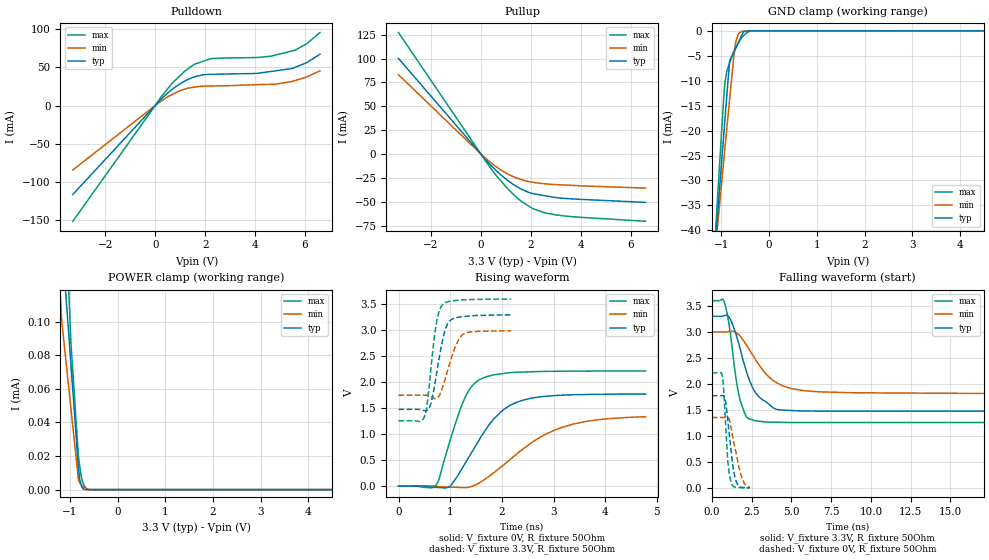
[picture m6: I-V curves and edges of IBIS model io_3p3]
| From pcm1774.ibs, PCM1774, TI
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|   io_3p3 Model
[Model]   io_3p3
Model_type   I/O
Polarity   Non-Inverting
Enable   Active-Low
Vinl = 0.99
Vinh = 2.31
Vmeas = 1.65
Vref = 1.65
Cref = 10pF
Rref = 50
|   typ   min   max
|   (nom PVT)   (fast PVT)   (slow PVT)
C_comp   8.631e-13   8.443e-13   8.826e-13
|ON state : BUFFER OUTPUT TURNED HIGH
|C_comp   8.631e-13   8.443e-13   8.826e-13
|OFF state: BUFFER IN HIGH IMPEDANCE
|C_comp   8.663e-13   8.474e-13   8.760e-13
| Where nom  PVT is Nominal Process, 3.3V, 26C
|   Fast PVT is Strong Process,  3.6V, -40C
|   Slow PVT is Weak Process,   3V, 86C
[Model Spec]
|Subparameter   typ   min   max
Vinh   2.31   2.1   2.52
Vinl   0.99   0.9   1.08
[Voltage Range]   3.3   3   3.6
|Ambient Temperature   25   85   -40
|Junction Temperature
[Temperature Range]   26   86   -40
[Pullup Reference]   3.3   3   3.6
[Pulldown Reference]   0   0   0
[Power Clamp Reference]   3.3   3   3.6
[GND Clamp Reference]   0   0   0
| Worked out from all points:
|   slope of the pulldown table from 0 to 0.495 V, typ, clamps not added: 30.8 ohm
|   slope of the pullup table from 0 to 0.495 V, typ, clamps not added: 34.8 ohm
|   GND clamp passes 1 mA (typ) near -0.58 V on its own axis
|   POWER clamp passes 1 mA (typ) near -2.56 V on its own axis
|   falling waveform, V_fixture 3.3V, R_fixture 50Ohm: 20-80 % time 1.19ns typ, 2.04ns min, 657ps max; typ from 3.3 V to 1.48 V
|   rising waveform, V_fixture 0V, R_fixture 50Ohm: 20-80 % time 730ps typ, 1.15ns min, 453ps max; typ from 0 V to 1.77 V
|   rising waveform, V_fixture 3.3V, R_fixture 50Ohm: 20-80 % time 201ps typ, 244ps min, 160ps max; typ from 1.48 V to 3.29 V
|   falling waveform, V_fixture 0V, R_fixture 50Ohm: 20-80 % time 394ps typ, 553ps min, 260ps max; typ from 1.77 V to 0.003 V
[Pulldown]
|   Voltage   I(typ)   I(min)   I(max)
-3.3V     -116.5mA   -84.42mA   -151.6mA
271.2mV   9.421mA    6.375mA    12.76mA
714mV     22.1mA     15.03mA    30.35mA
1.355V    34.85mA    23mA       49.31mA
1.589V    37.79mA    24.19mA    54.3mA
1.917V    40.27mA    25.38mA    57.97mA
2.222V    40.84mA    25.66mA    61.38mA
4.138V    42.37mA    27.45mA    62.98mA
4.8V      45.41mA    28mA       66.04mA
5.606V    50.05mA    32.82mA    72.53mA
6.082V    56.53mA    37.71mA    81.29mA
6.6V      67.25mA    45.42mA    95.62mA
[GND Clamp]
|   Voltage   I(typ)   I(min)   I(max)
-3.3V     -316.9mA   -268mA     -391.9mA
-1.111V   -40.79mA   -42.24mA   -38.36mA
-1.018V   -29.09mA   -32.77mA   -23.56mA
-949.2mV  -20.65mA   -25.85mA   -13.18mA
-920.4mV  -17.15mA   -22.94mA   -10.06mA
-825mV    -5.93mA    -13.45mA   -6.269mA
-738mV    -4.2mA     -5.003mA   -4.306mA
-702mV    -3.484mA   -2.489mA   -3.5mA
-648mV    -2.41mA    -754uA     -2.54mA
-567mV    -798.9uA   -93.27uA   -1.299mA
-243.6mV  -1.294uA   -116.1nA   -293.8nA
6.6V      0A         0A         0A
[Pullup]
|   Voltage   I(typ)   I(min)   I(max)
-3.3V     100.1mA    83.05mA    127.2mA
3mV       -185.6uA   -161.8uA   -246.1uA
363mV     -10.77mA   -8.423mA   -13.7mA
638.4mV   -18mA      -13.71mA   -23.32mA
1.103V    -28.28mA   -21.31mA   -37.21mA
1.643V    -37.09mA   -26.87mA   -49.95mA
2.064V    -41.39mA   -29.49mA   -56.97mA
2.525V    -43.47mA   -31.08mA   -61.32mA
3.018V    -45.7mA    -32.05mA   -63.8mA
3.983V    -47.45mA   -33.25mA   -66.26mA
6.6V      -50.64mA   -35.68mA   -70.46mA
[POWER Clamp]
|   Voltage   I(typ)   I(min)   I(max)
-3.3V     2.453mA    1.841mA    2.082mA
-1.947V   666.7uA    483.9uA    905uA
-1.178V   152uA      103.5uA    226.7uA
-1.165V   147uA      98.22uA    216.4uA
-981.6mV  75.07uA    48.64uA    88.02uA
-822mV    12.95uA    5.545uA    19.56uA
-788.7mV  5.054uA    3.952uA    12.72uA
-765.6mV  2.875uA    2.846uA    7.967uA
-736.8mV  979nA      2.084uA    4.528uA
-706.2mV  0A         1.47uA     2.727uA
-614.4mV  0A         0A         31.31nA
6.6V      0A         0A         0A
[Ramp]
R_load = 50
|   typ   min   max
dV/dt_r   1.06378/7.29577e-10   0.812608/1.17719e-09   1.32828/4.52863e-10
dV/dt_f   1.09414/1.19156e-09   0.751811/2.05432e-09   1.40532/6.56827e-10
[Falling Waveform]
V_fixture = 3.3V
V_fixture_min = 3V
V_fixture_max = 3.6V
R_fixture = 50Ohm
|   Time   V(typ)   V(min)   V(max)
0s        3.3V       3V         3.6V
770.7ps   3.31V      3V         3.581V
1.174ns   3.234V     3.015V     2.947V
1.504ns   2.966V     2.996V     2.133V
1.763ns   2.69V      2.921V     1.703V
2.146ns   2.264V     2.76V      1.384V
2.666ns   1.872V     2.508V     1.296V
4.032ns   1.515V     2.03V      1.263V
6.027ns   1.48V      1.864V     1.258V
27.16ns   1.477V     1.751V     1.258V
[Rising Waveform]
V_fixture = 0V
V_fixture_min = 0V
V_fixture_max = 0V
R_fixture = 50Ohm
|   Time   V(typ)   V(min)   V(max)
0s        476.9pV    717.9pV    417.6pV
739.7ps   -24.77mV   -3.221mV   36.69mV
1.015ns   14.61mV    -19.8mV    931.4mV
1.285ns   430.8mV    -29.7mV    1.697V
1.448ns   702.5mV    6.756mV    1.954V
1.653ns   1.034V     120mV      2.087V
2.04ns    1.475V     412.3mV    2.168V
2.528ns   1.683V     800.6mV    2.198V
3.379ns   1.757V     1.193V     2.211V
4.783ns   1.771V     1.336V     2.213V
[Rising Waveform]
V_fixture = 3.3V
V_fixture_min = 3V
V_fixture_max = 3.6V
R_fixture = 50Ohm
|   Time   V(typ)   V(min)   V(max)
0s        1.476V     1.747V     1.258V
504.4ps   1.45V      1.75V      1.344V
562.3ps   1.465V     1.745V     1.641V
619.5ps   1.566V     1.726V     2.178V
713.6ps   2.024V     1.683V     3.02V
770.7ps   2.369V     1.716V     3.312V
854.7ps   2.818V     1.908V     3.493V
984.7ps   3.173V     2.339V     3.553V
1.25ns    3.262V     2.922V     3.582V
2.178ns   3.295V     2.99V      3.597V
[Falling Waveform]
V_fixture = 0V
V_fixture_min = 0V
V_fixture_max = 0V
R_fixture = 50Ohm
|   Time   V(typ)   V(min)   V(max)
0s        1.773V     1.354V     2.214V
663ps     1.776V     1.354V     2.142V
739.7ps   1.775V     1.354V     1.892V
838.6ps   1.703V     1.357V     1.371V
1.006ns   1.284V     1.355V     504.6mV
1.216ns   696.1mV    1.142V     106.3mV
1.386ns   299.6mV    862.1mV    23.29mV
1.621ns   63.13mV    524.6mV    10.55mV
1.946ns   10.05mV    148.9mV    3.201mV
2.391ns   3.063mV    12.57mV    2.198mV
